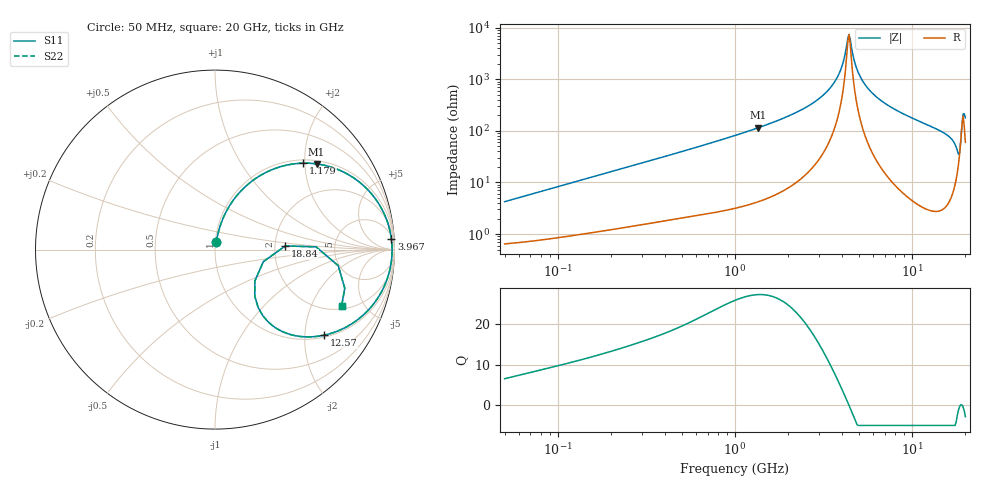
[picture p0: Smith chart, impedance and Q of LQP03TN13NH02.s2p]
!Murata Part Number: LQP03TN13NH02
!These Parameters are Measured in Series Mode Connection
!  o--[Z]--o
!Port1  Port2
!  o-------o
!Freq. Start=50[MHz] Stop=20[GHz], 401[Steps]
# Hz S RI R 50
!Freq.(Hz) S11(Real) S11(Imag) S21(Real) S21(Imag) S12(Real) S12(Imag) S22(Real) S22(Imag)
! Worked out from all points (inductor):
!   401 points, 50 MHz to 20 GHz, reference 50 ohm
!   read as one part in series: L = 13.3 nH near 51.52 MHz
!   highest Q = 27.2 at 1.349 GHz (marker M1), where L = 13.5 nH
!   self-resonance near 4.34 GHz
!   S11 on the Smith chart (normalised r, x): 50 MHz: 1.01, +0.08; 1.179 GHz: 1.07, +1.96; 3.967 GHz: 8, +31; 12.57 GHz: 1.06, -2.51; 18.84 GHz: 2.28, +0.11; 20 GHz: 2.20, -3.39
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5e7  0.00812 0.0413  0.9919 -0.0413  0.9919 -0.0413  0.00812 0.0413
1.364002e8  0.0217 0.1078  0.9783 -0.1078  0.9783 -0.1078  0.0217 0.1078
3.721004e8  0.0936 0.2636  0.9064 -0.2636  0.9064 -0.2636  0.0936 0.2636
1e9  0.4031 0.4715  0.5969 -0.4715  0.5969 -0.4715  0.4031 0.4715
1.179116e9  0.4906 0.4816  0.5094 -0.4816  0.5094 -0.4816  0.4906 0.4816
1.349283e9  0.5663 0.4776  0.4337 -0.4776  0.4337 -0.4776  0.5663 0.4776
1.99176e9  0.7784 0.3956  0.2216 -0.3956  0.2216 -0.3956  0.7784 0.3956
2.728004e9  0.9079 0.2624  0.0921 -0.2624  0.0921 -0.2624  0.9079 0.2624
3.466789e9  0.9665 0.1358  0.0335 -0.1358  0.0335 -0.1358  0.9665 0.1358
3.967106e9  0.9827 0.0596  0.0173 -0.0596  0.0173 -0.0596  0.9827 0.0596
4.275624e9  0.9864 0.0164  0.0136 -0.0164  0.0136 -0.0164  0.9864 0.0164
4.405649e9  0.9867 -0.000905  0.0133 0.000905  0.0133 0.000905  0.9867 -0.000905
4.539627e9  0.9865 -0.0183  0.0135 0.0183  0.0135 0.0183  0.9865 -0.0183
4.81993e9  0.9841 -0.0529  0.0159 0.0529  0.0159 0.0529  0.9841 -0.0529
5.273168e9  0.976 -0.1047  0.024 0.1047  0.024 0.1047  0.976 -0.1047
6.125241e9  0.9497 -0.1891  0.0503 0.1891  0.0503 0.1891  0.9497 -0.1891
7.442007e9  0.892 -0.2916  0.108 0.2916  0.108 0.2916  0.892 -0.2916
1.257102e10  0.6084 -0.4768  0.3916 0.4768  0.3916 0.4768  0.6084 -0.4768
1.670968e10  0.338 -0.4362  0.662 0.4362  0.662 0.4362  0.338 -0.4362
1.800918e10  0.2217 -0.2604  0.7783 0.2604  0.7783 0.2604  0.2217 -0.2604
1.88369e10  0.3917 0.0204  0.6083 -0.0204  0.6083 -0.0204  0.3917 0.0204
2e10  0.7058 -0.312  0.2942 0.312  0.2942 0.312  0.7058 -0.312
